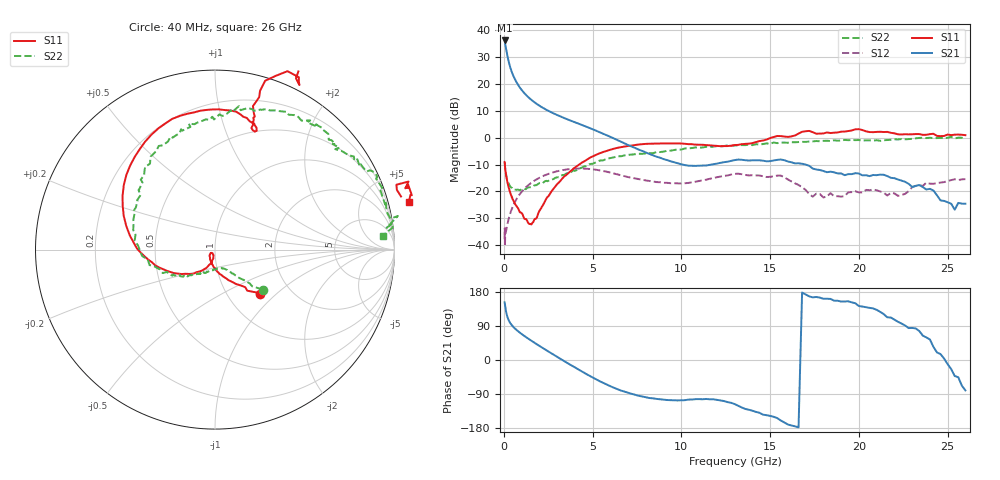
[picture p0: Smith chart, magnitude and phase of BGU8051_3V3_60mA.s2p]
! BGU8051_3V3_60mA
! Date/time Tue Jun 16 11:13:39 2015
! VAR V_out= 3.3000
! VAR I_out= 59.9900
! VAR V_in= 6.8030
! VAR I_in= 0.8789
# MHz S MA R 50
!  Freq-MHz  S11-mag  S11-arg  S21-mag  S21-arg  S12-mag  S12-arg  S22-mag  S22-arg
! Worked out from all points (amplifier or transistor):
!   197 points, 40 MHz to 26 GHz, reference 50 ohm
!   highest |S21| = 36.1 dB at 40 MHz (marker M1)
!   |S21| within 3 dB of that: start of sweep to 119.8 MHz
!   unconditionally stable (mu >= 1): 58.48 MHz to 62.87 MHz; 316.9 MHz to 12.98 GHz
!   at 800 MHz: K = 1.02, MAG = 19.9 dB, |S12| = -21.9 dB
!   at 6.4 GHz: K = 1.33, MAG = 2.9 dB, |S12| = -13.6 dB
!   at 26 GHz: K = -1.49, MSG = -4.6 dB, |S12| = -15.4 dB
!   lowest NFmin = 0.39 dB at 400 MHz
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40  0.3518 -45.0  63.97 152.2  0.01299 34.3  0.3472 -40.2
60  0.2905 -51.9  59.32 145.4  0.009611 13.8  0.2913 -44.6
80  0.2544 -53.0  53.89 139.2  0.01541 37.3  0.2528 -45.3
100  0.2242 -58.6  49.29 133.4  0.01716 40.3  0.2249 -47.4
120  0.2044 -61.9  45.25 128.2  0.01824 43.7  0.2078 -49.5
160  0.1712 -68.9  38.15 119.8  0.02126 51.4  0.1807 -51.9
200  0.1459 -75.7  32.64 113.4  0.02507 55.3  0.1614 -54.8
260  0.1216 -84.8  26.65 106.0  0.03028 58.3  0.1419 -57.5
320  0.102 -90.8  22.35 100.5  0.03554 60.9  0.1294 -60.1
400  0.08537 -99.3  18.31 94.7  0.04335 61.7  0.1204 -63.3
500  0.07113 -107.1  14.91 88.9  0.05284 62.1  0.1138 -68.6
700  0.05396 -120.4  10.85 79.8  0.0711 60.7  0.1074 -75.3
900  0.04103 -133.4  8.523 72.1  0.08944 57.4  0.1054 -83.9
1550  0.02432 -124.0  5.026 50.7  0.145 44.1  0.1213 -103.7
2700  0.1021 -113.2  2.923 16.9  0.2226 17.5  0.1669 -127.3
4400  0.3447 -165.2  1.714 -30.4  0.2663 -22.4  0.2777 -148.6
6400  0.6466 139.7  0.9001 -77.1  0.2081 -58.6  0.4504 173.9
8800  0.7781 96.0  0.4232 -103.7  0.1482 -70.3  0.5394 141.5
13200  0.7332 73.3  0.3916 -120.9  0.2139 -98.5  0.7224 95.2
17400  1.262 46.1  0.2661 165.2  0.07999 -149.3  0.8516 64.9
21800  1.23 20.8  0.1793 112.1  0.0938 -146.2  0.912 35.2
26000  1.111 13.7  0.05911 -80.2  0.1695 -175.8  0.9375 4.8
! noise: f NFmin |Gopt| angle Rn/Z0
400  0.3852  0.00546  11.13  0.0532
550  0.3944  0.02373  178.9  0.0517
950  0.4316  0.08894  184.2  0.049
1250  0.4712  0.1276  187.3  0.0481
1600  0.5303  0.1637  191.2  0.0485
1900  0.5919  0.1886  194.9  0.0501
2250  0.6766  0.2125  199.7  0.0537
2600  0.7751  0.233  204.7  0.0592
3300  1.013  0.2716  215  0.0767
4000  1.307  0.3161  223.7  0.1038
